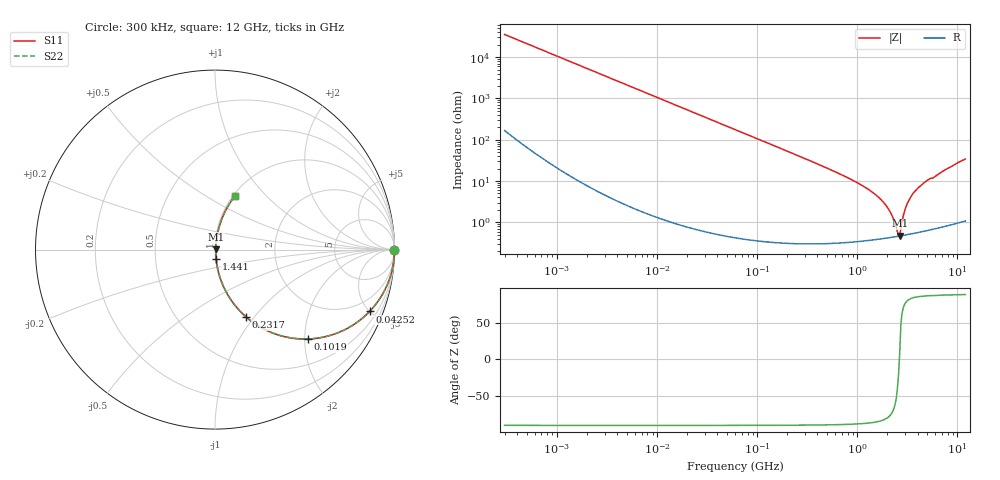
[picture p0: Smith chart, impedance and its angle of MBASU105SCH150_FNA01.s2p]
! MBASU105SCH150_FNA01  S-PARAMETER MODEL  ( General Type )
! Model Generated by TAIYO YUDEN Corporation (http://www.ty-top.com)
! Version 1.0
! TAIYO YUDEN Control No. 130207
! Copyright(c) 2013 TAIYO YUDEN CO.,LTD. All Rights Reserved.
! Product Description (link to TY-COMPAS)
! https://ds.yuden.co.jp/TYCOMPAS/or/detail?pn=MBASU105SCH150JFNA01&u=M
! Products Name : Multilayer Ceramic Capacitors
! Characteristics :
!  Capacitance : 15 pF , Rated Voltage : 50V , TCC : CH / C0H
!  Case Size : 1.0 x 0.5 / 0.039 x 0.02 [mm/inch] , Thickness : 0.5 / 0.02 [mm/inch]
!  (Conditions: Temperature = 25 degC , DC Bias Current/Voltage = 0A / 0V)
! External Node Assignments :
!  1  o---| |---o  2
! GND o---------o GND
! Frequency Range : 300000Hz  -  12GHz  [ 401 STEP ]
# MHz S RI R 50
! Freq[MHz].  S11 Real  S11 Imag  S21 Real  S21 Imag  S12 Real  S12 Imag  S22 Real  S22 Imag
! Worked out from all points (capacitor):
!   401 points, 300 kHz to 12 GHz, reference 50 ohm
!   read as one part in series: C = 15 pF near 316.3 kHz
!   lowest |Z| = 474 mohm at 2.651 GHz (marker M1)
!   series resonance near 2.629 GHz, so ESL is about 240 pH
!   S11 on the Smith chart (normalised r, x): 300 kHz: open; 42.52 MHz: 1.01, -5.00; 101.9 MHz: 1.01, -2.08; 231.7 MHz: 1.01, -0.91; 1.441 GHz: 1.01, -0.10; 12 GHz: 1.02, +0.68
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0.3  1 -0.00282  2.13e-05 0.00282  2.13e-05 0.00282  1 -0.00282
1.769972  0.9997 -0.0167  0.000303 0.0167  0.000303 0.0167  0.9997 -0.0167
10.44266  0.9903 -0.0973  0.00969 0.0973  0.00969 0.0973  0.9903 -0.0973
23.73947  0.9521 -0.2127  0.0479 0.2127  0.0479 0.2127  0.9521 -0.2127
42.51912  0.8614 -0.3446  0.1386 0.3446  0.1386 0.3446  0.8614 -0.3446
60  0.7574 -0.4275  0.2426 0.4275  0.2426 0.4275  0.7574 -0.4275
101.9188  0.5199 -0.4979  0.4801 0.4979  0.4801 0.4979  0.5199 -0.4979
231.6935  0.1731 -0.375  0.8269 0.375  0.8269 0.375  0.1731 -0.375
353.9943  0.0822 -0.2696  0.9178 0.2696  0.9178 0.2696  0.0822 -0.2696
848.5281  0.0156 -0.1101  0.9844 0.1101  0.9844 0.1101  0.0156 -0.1101
1441.349  0.00638 -0.0512  0.9936 0.0512  0.9936 0.0512  0.00638 -0.0512
1781.601  0.00504 -0.0321  0.995 0.0321  0.995 0.0321  0.00504 -0.0321
2088.533  0.00459 -0.0188  0.9954 0.0188  0.9954 0.0188  0.00459 -0.0188
2261.293  0.00452 -0.0123  0.9955 0.0123  0.9955 0.0123  0.00452 -0.0123
2514.07  0.00457 -0.00369  0.9954 0.00369  0.9954 0.00369  0.00457 -0.00369
2650.866  0.00466 0.000765  0.9953 -0.000765  0.9953 -0.000765  0.00466 0.000765
2947.191  0.00516 0.0171  0.9948 -0.0171  0.9948 -0.0171  0.00516 0.0171
3107.553  0.00564 0.0255  0.9944 -0.0255  0.9944 -0.0255  0.00564 0.0255
3454.93  0.00702 0.0422  0.993 -0.0422  0.993 -0.0422  0.00702 0.0422
3841.137  0.00903 0.0591  0.991 -0.0591  0.991 -0.0591  0.00903 0.0591
5140.631  0.0179 0.1063  0.9821 -0.1063  0.9821 -0.1063  0.0179 0.1063
12000  0.1121 0.3001  0.8879 -0.3001  0.8879 -0.3001  0.1121 0.3001
